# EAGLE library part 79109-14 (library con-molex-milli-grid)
RECEPTACAL
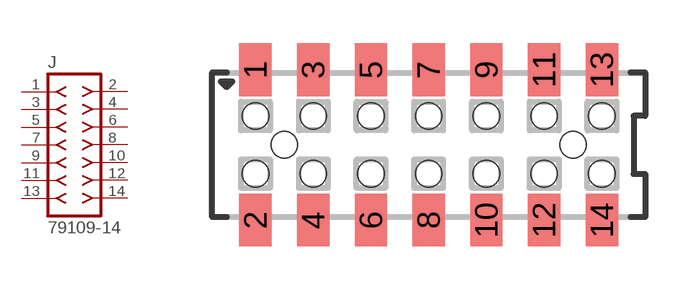
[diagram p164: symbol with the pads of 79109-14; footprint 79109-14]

Designator prefix J

## 79109-14  [79109-14]
1  1  pas
2  2  pas
3  3  pas
4  4  pas
5  5  pas
6  6  pas
7  7  pas
8  8  pas
9  9  pas
10  10  pas
11  11  pas
12  12  pas
13  13  pas
14  14  pas

## Footprint 79109-14 (pad centres in mm)
RECEPTACAL SMD Dual Row, Vertical, Pass-Thru
smd 1.12 x 1.83: 1 -6,2.6; 2 -6,-2.6; 3 -4,2.6; 4 -4,-2.6; 5 -2,2.6; 6 -2,-2.6; 7 0,2.6; 8 0,-2.6; 9 2,2.6; 10 2,-2.6; 11 4,2.6; 12 4,-2.6; 13 6,2.6; 14 6,-2.6
hole 0.914 at -5,0
hole 0.914 at -6,1
hole 0.914 at -6,-1
hole 0.914 at -4,-1
hole 0.914 at -4,1
hole 0.914 at -2,-1
hole 0.914 at -2,1
hole 0.914 at 5,0
hole 0.914 at 0,1
hole 0.914 at 0,-1
hole 0.914 at 2,1
hole 0.914 at 2,-1
hole 0.914 at 4,1
hole 0.914 at 4,-1
hole 0.914 at 6,1
hole 0.914 at 6,-1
